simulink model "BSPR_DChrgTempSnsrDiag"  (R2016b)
settings: Solver=FixedStepDiscrete  StartTime=0.0  StopTime=10.0  FixedStep=0.02  RelTol=1e-3  EnableMultiTasking=on
undefined symbols (not defined in the file): BCCR_cntDChrgTempDiag_CW, bin2dec, BSPR_tiDChrgTNegElecMax_C, BSPR_tiDChrgTNegElecMin_C, BSPR_tiDChrgTNegJit_C, BSPR_tiDChrgTNegVld_C, BSPR_tiDChrgTPosElecMax_C, BSPR_tiDChrgTPosElecMin_C, BSPR_tiDChrgTPosJit_C, BSPR_tiDChrgTPosVld_C, BSPR_uDChrgTNegElecMax_C, BSPR_uDChrgTNegElecMin_C, BSPR_uDChrgTNegJitDiff_C, BSPR_uDChrgTPosElecMax_C, BSPR_uDChrgTPosElecMin_C, BSPR_uDChrgTPosJitDiff_C
libraries: simulink x48

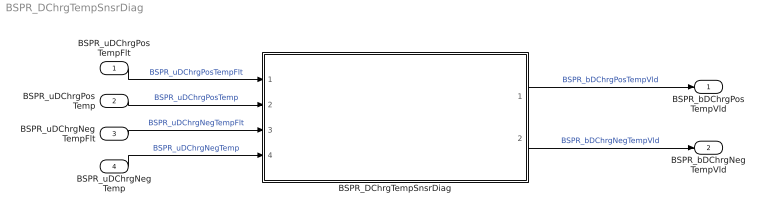
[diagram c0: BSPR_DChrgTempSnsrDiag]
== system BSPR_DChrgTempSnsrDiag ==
  BSPR_uDChrgPosTempFlt : Inport
  BSPR_uDChrgPosTemp : Inport  Port=2
  BSPR_uDChrgNegTempFlt : Inport  Port=3
  BSPR_uDChrgNegTemp : Inport  Port=4
  BSPR_DChrgTempSnsrDiag : Subsystem
  BSPR_bDChrgPosTempVld : Outport
  BSPR_bDChrgNegTempVld : Outport  Port=2
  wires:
  BSPR_uDChrgPosTempFlt/1 -> BSPR_DChrgTempSnsrDiag/1(BSPR_uDChrgPosTempFlt)  "BSPR_uDChrgPosTempFlt"
  BSPR_uDChrgPosTemp/1 -> BSPR_DChrgTempSnsrDiag/2(BSPR_uDChrgPosTemp)  "BSPR_uDChrgPosTemp"
  BSPR_uDChrgNegTempFlt/1 -> BSPR_DChrgTempSnsrDiag/3(BSPR_uDChrgNegTempFlt)  "BSPR_uDChrgNegTempFlt"
  BSPR_uDChrgNegTemp/1 -> BSPR_DChrgTempSnsrDiag/4(BSPR_uDChrgNegTemp)  "BSPR_uDChrgNegTemp"
  BSPR_DChrgTempSnsrDiag/1(BSPR_bDChrgPosTempVld) -> BSPR_bDChrgPosTempVld/1  "BSPR_bDChrgPosTempVld"
  BSPR_DChrgTempSnsrDiag/2(BSPR_bDChrgNegTempVld) -> BSPR_bDChrgNegTempVld/1  "BSPR_bDChrgNegTempVld"

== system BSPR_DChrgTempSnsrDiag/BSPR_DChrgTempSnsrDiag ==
  BSPR_uDChrgPosTempFlt : Inport
  BSPR_uDChrgPosTemp : Inport  Port=2
  BSPR_uDChrgNegTempFlt : Inport  Port=3
  BSPR_uDChrgNegTemp : Inport  Port=4
  DChrgTNegErrChk : Subsystem
  DChrgTPosErrChk : Subsystem
  DChrgTempDsmRpt : Subsystem
  BSPR_bDChrgPosTempVld : Outport
  BSPR_bDChrgNegTempVld : Outport  Port=2
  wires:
  BSPR_uDChrgPosTempFlt/1 -> DChrgTPosErrChk/1(BSPR_uDChrgPosTempFlt)
  BSPR_uDChrgPosTemp/1 -> DChrgTPosErrChk/2(BSPR_uDChrgPosTemp)
  DChrgTPosErrChk/1(BSPR_bDChrgTPosJitErrStt) -> DChrgTempDsmRpt/1(BSPR_bDChrgTPosJitErrStt)
  DChrgTPosErrChk/2(BSPR_bDChrgTPosMaxErrStt) -> DChrgTempDsmRpt/2(BSPR_bDChrgTPosMaxErrStt)
  DChrgTPosErrChk/3(BSPR_bDChrgTPosMinErrStt) -> DChrgTempDsmRpt/3(BSPR_bDChrgTPosMinErrStt)
  DChrgTPosErrChk/4(BSPR_bDChrgTPosJitErrDet) -> DChrgTempDsmRpt/4(BSPR_bDChrgTPosJitErrDet)
  DChrgTPosErrChk/5(BSPR_bDChrgTPosJitErrHeal) -> DChrgTempDsmRpt/5(BSPR_bDChrgTPosJitErrHeal)
  DChrgTPosErrChk/6(BSPR_bDChrgTPosMaxErrDet) -> DChrgTempDsmRpt/6(BSPR_bDChrgTPosMaxErrDet)
  DChrgTPosErrChk/7(BSPR_bDChrgTPosMaxErrHeal) -> DChrgTempDsmRpt/7(BSPR_bDChrgTPosMaxErrHeal)
  DChrgTPosErrChk/8(BSPR_bDChrgTPosMinErrDet) -> DChrgTempDsmRpt/8(BSPR_bDChrgTPosMinErrDet)
  DChrgTPosErrChk/9(BSPR_bDChrgTPosMinErrHeal) -> DChrgTempDsmRpt/9(BSPR_bDChrgTPosMinErrHeal)
  DChrgTempDsmRpt/1(BSPR_bDChrgPosTempVld) -> BSPR_bDChrgPosTempVld/1
  BSPR_uDChrgNegTempFlt/1 -> DChrgTNegErrChk/1(BSPR_uDChrgNegTempFlt)
  BSPR_uDChrgNegTemp/1 -> DChrgTNegErrChk/2(BSPR_uDChrgNegTemp)
  DChrgTempDsmRpt/2(BSPR_bDChrgNegTempVld) -> BSPR_bDChrgNegTempVld/1
  DChrgTNegErrChk/1(BSPR_bDChrgTNegJitErrStt) -> DChrgTempDsmRpt/10(BSPR_bDChrgTNegJitErrStt)
  DChrgTNegErrChk/2(BSPR_bDChrgTNegMaxErrStt) -> DChrgTempDsmRpt/11(BSPR_bDChrgTNegMaxErrStt)
  DChrgTNegErrChk/3(BSPR_bDChrgTNegMinErrStt) -> DChrgTempDsmRpt/12(BSPR_bDChrgTNegMinErrStt)
  DChrgTNegErrChk/4(BSPR_bDChrgTNegJitErrDet) -> DChrgTempDsmRpt/13(BSPR_bDChrgTNegJitErrDet)
  DChrgTNegErrChk/5(BSPR_bDChrgTNegJitErrHeal) -> DChrgTempDsmRpt/14(BSPR_bDChrgTNegJitErrHeal)
  DChrgTNegErrChk/6(BSPR_bDChrgTNegMaxErrDet) -> DChrgTempDsmRpt/15(BSPR_bDChrgTNegMaxErrDet)
  DChrgTNegErrChk/7(BSPR_bDChrgTNegMaxErrHeal) -> DChrgTempDsmRpt/16(BSPR_bDChrgTNegMaxErrHeal)
  DChrgTNegErrChk/8(BSPR_bDChrgTNegMinErrDet) -> DChrgTempDsmRpt/17(BSPR_bDChrgTNegMinErrDet)
  DChrgTNegErrChk/9(BSPR_bDChrgTNegMinErrHeal) -> DChrgTempDsmRpt/18(BSPR_bDChrgTNegMinErrHeal)

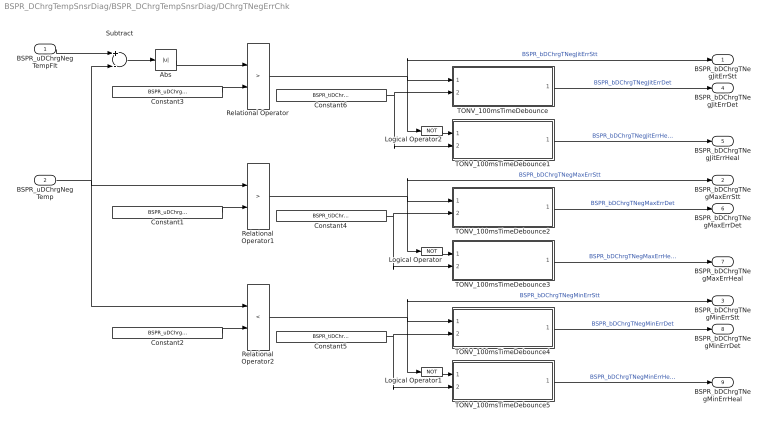
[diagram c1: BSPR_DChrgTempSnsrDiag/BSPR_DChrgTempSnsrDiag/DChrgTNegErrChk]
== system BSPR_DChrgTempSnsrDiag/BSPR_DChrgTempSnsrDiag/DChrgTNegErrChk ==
  BSPR_uDChrgNegTempFlt : Inport
  BSPR_uDChrgNegTemp : Inport  Port=2
  Abs : Abs
  Constant1 : Constant  Value=BSPR_uDChrgTNegElecMax_C  OutDataTypeStr=single
  Constant2 : Constant  Value=BSPR_uDChrgTNegElecMin_C  OutDataTypeStr=single
  Constant3 : Constant  Value=BSPR_uDChrgTNegJitDiff_C  OutDataTypeStr=single
  Constant4 : Constant  Value=BSPR_tiDChrgTNegElecMax_C  OutDataTypeStr=single
  Constant5 : Constant  Value=BSPR_tiDChrgTNegElecMin_C  OutDataTypeStr=single
  Constant6 : Constant  Value=BSPR_tiDChrgTNegJit_C  OutDataTypeStr=single
  Logical Operator : Logic  Operator=NOT  AllPortsSameDT=off  OutDataTypeStr=boolean
  Logical Operator1 : Logic  Operator=NOT  AllPortsSameDT=off  OutDataTypeStr=boolean
  Logical Operator2 : Logic  Operator=NOT  AllPortsSameDT=off  OutDataTypeStr=boolean
  Relational Operator : RelationalOperator  Operator=>  OutDataTypeStr=boolean  RndMeth=Simplest
  Relational Operator1 : RelationalOperator  Operator=>  OutDataTypeStr=boolean  RndMeth=Simplest
  Relational Operator2 : RelationalOperator  Operator=<  OutDataTypeStr=boolean  RndMeth=Simplest
  Subtract : Sum  Inputs=+-
  TONV_100msTimeDebounce : Subsystem  TreatAsAtomicUnit=on  RTWFcnName=TONV_100msTimeDebounce  RTWFileName=SrvLib
  TONV_100msTimeDebounce1 : Subsystem  TreatAsAtomicUnit=on  RTWFcnName=TONV_100msTimeDebounce  RTWFileName=SrvLib
  TONV_100msTimeDebounce2 : Subsystem  TreatAsAtomicUnit=on  RTWFcnName=TONV_100msTimeDebounce  RTWFileName=SrvLib
  TONV_100msTimeDebounce3 : Subsystem  TreatAsAtomicUnit=on  RTWFcnName=TONV_100msTimeDebounce  RTWFileName=SrvLib
  TONV_100msTimeDebounce4 : Subsystem  TreatAsAtomicUnit=on  RTWFcnName=TONV_100msTimeDebounce  RTWFileName=SrvLib
  TONV_100msTimeDebounce5 : Subsystem  TreatAsAtomicUnit=on  RTWFcnName=TONV_100msTimeDebounce  RTWFileName=SrvLib
  BSPR_bDChrgTNegJitErrStt : Outport
  BSPR_bDChrgTNegMaxErrStt : Outport  Port=2
  BSPR_bDChrgTNegMinErrStt : Outport  Port=3
  BSPR_bDChrgTNegJitErrDet : Outport  Port=4
  BSPR_bDChrgTNegJitErrHeal : Outport  Port=5
  BSPR_bDChrgTNegMaxErrDet : Outport  Port=6
  BSPR_bDChrgTNegMaxErrHeal : Outport  Port=7
  BSPR_bDChrgTNegMinErrDet : Outport  Port=8
  BSPR_bDChrgTNegMinErrHeal : Outport  Port=9
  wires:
  TONV_100msTimeDebounce2/1(y) -> BSPR_bDChrgTNegMaxErrDet/1  "BSPR_bDChrgTNegMaxErrDet"
  TONV_100msTimeDebounce1/1(y) -> BSPR_bDChrgTNegJitErrHeal/1  "BSPR_bDChrgTNegJitErrHeal"
  TONV_100msTimeDebounce3/1(y) -> BSPR_bDChrgTNegMaxErrHeal/1  "BSPR_bDChrgTNegMaxErrHeal"
  TONV_100msTimeDebounce4/1(y) -> BSPR_bDChrgTNegMinErrDet/1  "BSPR_bDChrgTNegMinErrDet"
  Logical Operator/1 -> TONV_100msTimeDebounce3/1(u)
  Constant4/1 -> TONV_100msTimeDebounce3/2(T), TONV_100msTimeDebounce2/2(T)
  BSPR_uDChrgNegTemp/1 -> Relational Operator1/1, Relational Operator2/1, Subtract/2
  Relational Operator1/1 -> Logical Operator/1, TONV_100msTimeDebounce2/1(u), BSPR_bDChrgTNegMaxErrStt/1  "BSPR_bDChrgTNegMaxErrStt"
  Constant1/1 -> Relational Operator1/2
  Constant2/1 -> Relational Operator2/2
  Constant6/1 -> TONV_100msTimeDebounce1/2(T), TONV_100msTimeDebounce/2(T)
  Relational Operator/1 -> Logical Operator2/1, TONV_100msTimeDebounce/1(u), BSPR_bDChrgTNegJitErrStt/1  "BSPR_bDChrgTNegJitErrStt"
  BSPR_uDChrgNegTempFlt/1 -> Subtract/1
  Subtract/1 -> Abs/1
  Abs/1 -> Relational Operator/1
  Constant3/1 -> Relational Operator/2
  TONV_100msTimeDebounce/1(y) -> BSPR_bDChrgTNegJitErrDet/1  "BSPR_bDChrgTNegJitErrDet"
  Constant5/1 -> TONV_100msTimeDebounce4/2(T), TONV_100msTimeDebounce5/2(T)
  Relational Operator2/1 -> TONV_100msTimeDebounce4/1(u), Logical Operator1/1, BSPR_bDChrgTNegMinErrStt/1  "BSPR_bDChrgTNegMinErrStt"
  TONV_100msTimeDebounce5/1(y) -> BSPR_bDChrgTNegMinErrHeal/1  "BSPR_bDChrgTNegMinErrHeal"
  Logical Operator1/1 -> TONV_100msTimeDebounce5/1(u)
  Logical Operator2/1 -> TONV_100msTimeDebounce1/1(u)

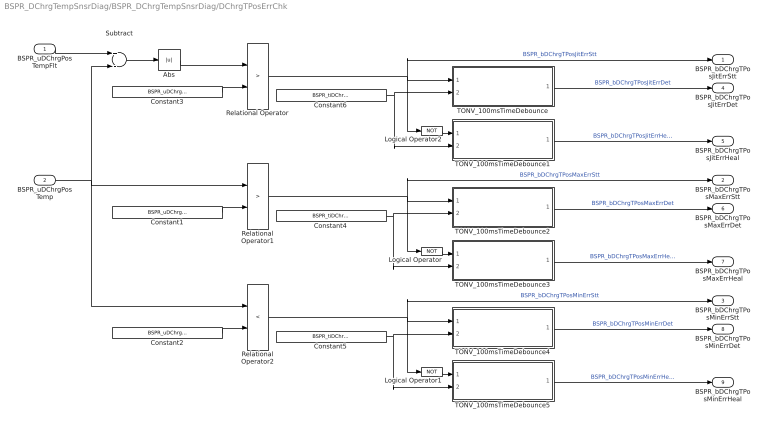
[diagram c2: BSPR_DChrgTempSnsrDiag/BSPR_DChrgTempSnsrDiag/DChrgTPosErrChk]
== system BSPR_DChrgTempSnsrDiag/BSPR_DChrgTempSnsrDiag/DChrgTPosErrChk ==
  BSPR_uDChrgPosTempFlt : Inport
  BSPR_uDChrgPosTemp : Inport  Port=2
  Abs : Abs
  Constant1 : Constant  Value=BSPR_uDChrgTPosElecMax_C  OutDataTypeStr=single
  Constant2 : Constant  Value=BSPR_uDChrgTPosElecMin_C  OutDataTypeStr=single
  Constant3 : Constant  Value=BSPR_uDChrgTPosJitDiff_C  OutDataTypeStr=single
  Constant4 : Constant  Value=BSPR_tiDChrgTPosElecMax_C  OutDataTypeStr=single
  Constant5 : Constant  Value=BSPR_tiDChrgTPosElecMin_C  OutDataTypeStr=single
  Constant6 : Constant  Value=BSPR_tiDChrgTPosJit_C  OutDataTypeStr=single
  Logical Operator : Logic  Operator=NOT  AllPortsSameDT=off  OutDataTypeStr=boolean
  Logical Operator1 : Logic  Operator=NOT  AllPortsSameDT=off  OutDataTypeStr=boolean
  Logical Operator2 : Logic  Operator=NOT  AllPortsSameDT=off  OutDataTypeStr=boolean
  Relational Operator : RelationalOperator  Operator=>  OutDataTypeStr=boolean  RndMeth=Simplest
  Relational Operator1 : RelationalOperator  Operator=>  OutDataTypeStr=boolean  RndMeth=Simplest
  Relational Operator2 : RelationalOperator  Operator=<  OutDataTypeStr=boolean  RndMeth=Simplest
  Subtract : Sum  Inputs=+-
  TONV_100msTimeDebounce : Subsystem  TreatAsAtomicUnit=on  RTWFcnName=TONV_100msTimeDebounce  RTWFileName=SrvLib
  TONV_100msTimeDebounce1 : Subsystem  TreatAsAtomicUnit=on  RTWFcnName=TONV_100msTimeDebounce  RTWFileName=SrvLib
  TONV_100msTimeDebounce2 : Subsystem  TreatAsAtomicUnit=on  RTWFcnName=TONV_100msTimeDebounce  RTWFileName=SrvLib
  TONV_100msTimeDebounce3 : Subsystem  TreatAsAtomicUnit=on  RTWFcnName=TONV_100msTimeDebounce  RTWFileName=SrvLib
  TONV_100msTimeDebounce4 : Subsystem  TreatAsAtomicUnit=on  RTWFcnName=TONV_100msTimeDebounce  RTWFileName=SrvLib
  TONV_100msTimeDebounce5 : Subsystem  TreatAsAtomicUnit=on  RTWFcnName=TONV_100msTimeDebounce  RTWFileName=SrvLib
  BSPR_bDChrgTPosJitErrStt : Outport
  BSPR_bDChrgTPosMaxErrStt : Outport  Port=2
  BSPR_bDChrgTPosMinErrStt : Outport  Port=3
  BSPR_bDChrgTPosJitErrDet : Outport  Port=4
  BSPR_bDChrgTPosJitErrHeal : Outport  Port=5
  BSPR_bDChrgTPosMaxErrDet : Outport  Port=6
  BSPR_bDChrgTPosMaxErrHeal : Outport  Port=7
  BSPR_bDChrgTPosMinErrDet : Outport  Port=8
  BSPR_bDChrgTPosMinErrHeal : Outport  Port=9
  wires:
  Logical Operator1/1 -> TONV_100msTimeDebounce5/1(u)
  TONV_100msTimeDebounce5/1(y) -> BSPR_bDChrgTPosMinErrHeal/1  "BSPR_bDChrgTPosMinErrHeal"
  Relational Operator2/1 -> BSPR_bDChrgTPosMinErrStt/1, Logical Operator1/1, TONV_100msTimeDebounce4/1(u)  "BSPR_bDChrgTPosMinErrStt"
  Constant5/1 -> TONV_100msTimeDebounce5/2(T), TONV_100msTimeDebounce4/2(T)
  TONV_100msTimeDebounce/1(y) -> BSPR_bDChrgTPosJitErrDet/1  "BSPR_bDChrgTPosJitErrDet"
  Constant3/1 -> Relational Operator/2
  Abs/1 -> Relational Operator/1
  Subtract/1 -> Abs/1
  BSPR_uDChrgPosTempFlt/1 -> Subtract/1
  Relational Operator/1 -> Logical Operator2/1, BSPR_bDChrgTPosJitErrStt/1, TONV_100msTimeDebounce/1(u)  "BSPR_bDChrgTPosJitErrStt"
  Constant6/1 -> TONV_100msTimeDebounce/2(T), TONV_100msTimeDebounce1/2(T)
  Constant2/1 -> Relational Operator2/2
  Constant1/1 -> Relational Operator1/2
  Relational Operator1/1 -> BSPR_bDChrgTPosMaxErrStt/1, TONV_100msTimeDebounce2/1(u), Logical Operator/1  "BSPR_bDChrgTPosMaxErrStt"
  BSPR_uDChrgPosTemp/1 -> Subtract/2, Relational Operator2/1, Relational Operator1/1
  Constant4/1 -> TONV_100msTimeDebounce2/2(T), TONV_100msTimeDebounce3/2(T)
  Logical Operator/1 -> TONV_100msTimeDebounce3/1(u)
  TONV_100msTimeDebounce4/1(y) -> BSPR_bDChrgTPosMinErrDet/1  "BSPR_bDChrgTPosMinErrDet"
  TONV_100msTimeDebounce3/1(y) -> BSPR_bDChrgTPosMaxErrHeal/1  "BSPR_bDChrgTPosMaxErrHeal"
  TONV_100msTimeDebounce1/1(y) -> BSPR_bDChrgTPosJitErrHeal/1  "BSPR_bDChrgTPosJitErrHeal"
  TONV_100msTimeDebounce2/1(y) -> BSPR_bDChrgTPosMaxErrDet/1  "BSPR_bDChrgTPosMaxErrDet"
  Logical Operator2/1 -> TONV_100msTimeDebounce1/1(u)

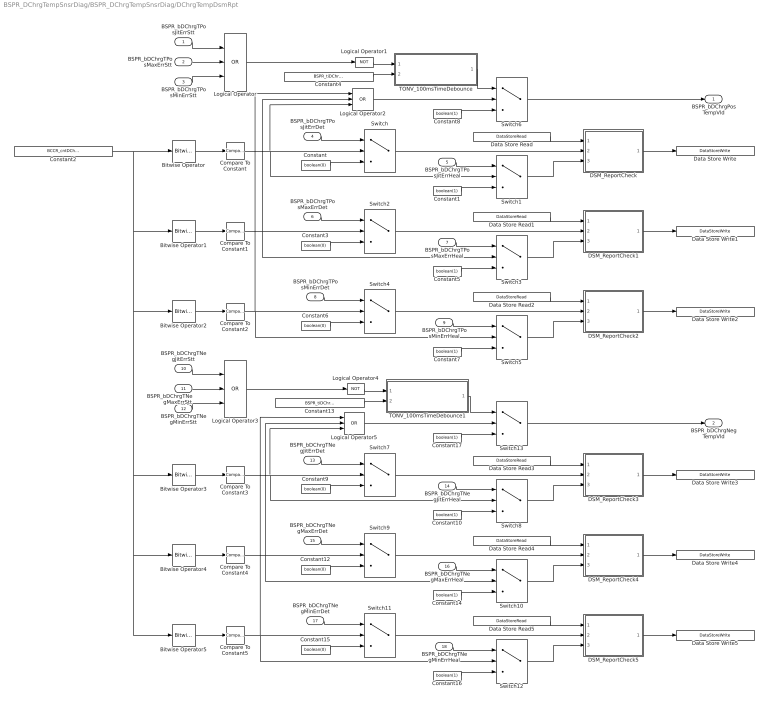
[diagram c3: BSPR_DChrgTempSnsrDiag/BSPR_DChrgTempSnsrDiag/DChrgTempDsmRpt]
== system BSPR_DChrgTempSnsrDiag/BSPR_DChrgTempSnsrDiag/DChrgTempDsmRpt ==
  BSPR_bDChrgTPosJitErrStt : Inport
  BSPR_bDChrgTPosMaxErrStt : Inport  Port=2
  BSPR_bDChrgTPosMinErrStt : Inport  Port=3
  BSPR_bDChrgTPosJitErrDet : Inport  Port=4
  BSPR_bDChrgTPosJitErrHeal : Inport  Port=5
  BSPR_bDChrgTPosMaxErrDet : Inport  Port=6
  BSPR_bDChrgTPosMaxErrHeal : Inport  Port=7
  BSPR_bDChrgTPosMinErrDet : Inport  Port=8
  BSPR_bDChrgTPosMinErrHeal : Inport  Port=9
  BSPR_bDChrgTNegJitErrStt : Inport  Port=10
  BSPR_bDChrgTNegMaxErrStt : Inport  Port=11
  BSPR_bDChrgTNegMinErrStt : Inport  Port=12
  BSPR_bDChrgTNegJitErrDet : Inport  Port=13
  BSPR_bDChrgTNegJitErrHeal : Inport  Port=14
  BSPR_bDChrgTNegMaxErrDet : Inport  Port=15
  BSPR_bDChrgTNegMaxErrHeal : Inport  Port=16
  BSPR_bDChrgTNegMinErrDet : Inport  Port=17
  BSPR_bDChrgTNegMinErrHeal : Inport  Port=18
  Bitwise Operator : simulink/Logic and Bit Operations/Bitwise Operator  logicop=AND  UseBitMask=on  BitMask=bin2dec('00000001')  BitMaskRealWorld=Stored Integer
  Bitwise Operator1 : simulink/Logic and Bit Operations/Bitwise Operator  logicop=AND  UseBitMask=on  BitMask=bin2dec('00000010')  BitMaskRealWorld=Stored Integer
  Bitwise Operator2 : simulink/Logic and Bit Operations/Bitwise Operator  logicop=AND  UseBitMask=on  BitMask=bin2dec('00000100')  BitMaskRealWorld=Stored Integer
  Bitwise Operator3 : simulink/Logic and Bit Operations/Bitwise Operator  logicop=AND  UseBitMask=on  BitMask=bin2dec('00001000')  BitMaskRealWorld=Stored Integer
  Bitwise Operator4 : simulink/Logic and Bit Operations/Bitwise Operator  logicop=AND  UseBitMask=on  BitMask=bin2dec('00010000')  BitMaskRealWorld=Stored Integer
  Bitwise Operator5 : simulink/Logic and Bit Operations/Bitwise Operator  logicop=AND  UseBitMask=on  BitMask=bin2dec('00100000')  BitMaskRealWorld=Stored Integer
  Compare To Constant : simulink/Logic and Bit Operations/Compare To Constant  relop===  const=1  OutDataTypeStr=boolean
  Compare To Constant1 : simulink/Logic and Bit Operations/Compare To Constant  relop===  const=2  OutDataTypeStr=boolean
  Compare To Constant2 : simulink/Logic and Bit Operations/Compare To Constant  relop===  const=4  OutDataTypeStr=boolean
  Compare To Constant3 : simulink/Logic and Bit Operations/Compare To Constant  relop===  const=8  OutDataTypeStr=boolean
  Compare To Constant4 : simulink/Logic and Bit Operations/Compare To Constant  relop===  const=16  OutDataTypeStr=boolean
  Compare To Constant5 : simulink/Logic and Bit Operations/Compare To Constant  relop===  const=32  OutDataTypeStr=boolean
  Constant{,3,6,9,12,15} (6 alike) : Constant  Value=boolean(0)  OutDataTypeStr=boolean
  Constant{1,5,7..8,10,14,16..17} (8 alike) : Constant  Value=boolean(1)  OutDataTypeStr=boolean
  Constant13 : Constant  Value=BSPR_tiDChrgTNegVld_C  OutDataTypeStr=single
  Constant2 : Constant  Value=BCCR_cntDChrgTempDiag_CW
  Constant4 : Constant  Value=BSPR_tiDChrgTPosVld_C  OutDataTypeStr=single
  DSM_ReportCheck : Subsystem  TreatAsAtomicUnit=on  RTWFcnName=DSM_ReportCheck  RTWFileName=SrvLib
  DSM_ReportCheck1 : Subsystem  TreatAsAtomicUnit=on  RTWFcnName=DSM_ReportCheck  RTWFileName=SrvLib
  DSM_ReportCheck2 : Subsystem  TreatAsAtomicUnit=on  RTWFcnName=DSM_ReportCheck  RTWFileName=SrvLib
  DSM_ReportCheck3 : Subsystem  TreatAsAtomicUnit=on  RTWFcnName=DSM_ReportCheck  RTWFileName=SrvLib
  DSM_ReportCheck4 : Subsystem  TreatAsAtomicUnit=on  RTWFcnName=DSM_ReportCheck  RTWFileName=SrvLib
  DSM_ReportCheck5 : Subsystem  TreatAsAtomicUnit=on  RTWFcnName=DSM_ReportCheck  RTWFileName=SrvLib
  Data Store Read : DataStoreRead  DataStoreName=DFC_DChrgTPosElecSig
  Data Store Read1 : DataStoreRead  DataStoreName=DFC_DChrgTPosElecMax
  Data Store Read2 : DataStoreRead  DataStoreName=DFC_DChrgTPosElecMin
  Data Store Read3 : DataStoreRead  DataStoreName=DFC_DChrgTNegElecSig
  Data Store Read4 : DataStoreRead  DataStoreName=DFC_DChrgTNegElecMax
  Data Store Read5 : DataStoreRead  DataStoreName=DFC_DChrgTNegElecMin
  Data Store Write : DataStoreWrite  DataStoreName=DFC_DChrgTPosElecSig
  Data Store Write1 : DataStoreWrite  DataStoreName=DFC_DChrgTPosElecMax
  Data Store Write2 : DataStoreWrite  DataStoreName=DFC_DChrgTPosElecMin
  Data Store Write3 : DataStoreWrite  DataStoreName=DFC_DChrgTNegElecSig
  Data Store Write4 : DataStoreWrite  DataStoreName=DFC_DChrgTNegElecMax
  Data Store Write5 : DataStoreWrite  DataStoreName=DFC_DChrgTNegElecMin
  Logical Operator{,2..3,5} (4 alike) : Logic  Operator=OR  Inputs=3  AllPortsSameDT=off  OutDataTypeStr=boolean
  Logical Operator1 : Logic  Operator=NOT  AllPortsSameDT=off  OutDataTypeStr=boolean
  Logical Operator4 : Logic  Operator=NOT  AllPortsSameDT=off  OutDataTypeStr=boolean
  Switch{,1..13} (14 alike) : Switch  Criteria=u2 > Threshold
  TONV_100msTimeDebounce : Subsystem  TreatAsAtomicUnit=on  RTWFcnName=TONV_100msTimeDebounce  RTWFileName=SrvLib
  TONV_100msTimeDebounce1 : Subsystem  TreatAsAtomicUnit=on  RTWFcnName=TONV_100msTimeDebounce  RTWFileName=SrvLib
  BSPR_bDChrgPosTempVld : Outport
  BSPR_bDChrgNegTempVld : Outport  Port=2
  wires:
  BSPR_bDChrgTPosJitErrStt/1 -> Logical Operator/1
  BSPR_bDChrgTPosMaxErrStt/1 -> Logical Operator/2
  BSPR_bDChrgTPosMinErrStt/1 -> Logical Operator/3
  Logical Operator/1 -> Logical Operator1/1
  Logical Operator1/1 -> TONV_100msTimeDebounce/1(u)
  Switch6/1 -> BSPR_bDChrgPosTempVld/1
  Constant4/1 -> TONV_100msTimeDebounce/2(T)
  Constant/1 -> Switch/3
  BSPR_bDChrgTPosJitErrDet/1 -> Switch/1
  BSPR_bDChrgTPosJitErrHeal/1 -> Switch1/1
  Constant1/1 -> Switch1/3
  Switch1/1 -> DSM_ReportCheck/3(Heal)
  Switch/1 -> DSM_ReportCheck/2(Err)
  Bitwise Operator/1 -> Compare To Constant/1
  Compare To Constant/1 -> Logical Operator2/3, Switch1/2, Switch/2
  Constant3/1 -> Switch2/3
  Constant5/1 -> Switch3/3
  Switch3/1 -> DSM_ReportCheck1/3(Heal)
  Switch2/1 -> DSM_ReportCheck1/2(Err)
  BSPR_bDChrgTPosMaxErrHeal/1 -> Switch3/1
  BSPR_bDChrgTPosMaxErrDet/1 -> Switch2/1
  Bitwise Operator1/1 -> Compare To Constant1/1
  Compare To Constant1/1 -> Switch2/2, Switch3/2, Logical Operator2/2
  Data Store Read1/1 -> DSM_ReportCheck1/1(Dfc_id_nv)
  Data Store Read/1 -> DSM_ReportCheck/1(Dfc_id_nv)
  Constant6/1 -> Switch4/3
  Constant7/1 -> Switch5/3
  Switch5/1 -> DSM_ReportCheck2/3(Heal)
  Switch4/1 -> DSM_ReportCheck2/2(Err)
  BSPR_bDChrgTPosMinErrHeal/1 -> Switch5/1
  BSPR_bDChrgTPosMinErrDet/1 -> Switch4/1
  Bitwise Operator2/1 -> Compare To Constant2/1
  Compare To Constant2/1 -> Switch4/2, Switch5/2, Logical Operator2/1
  Data Store Read2/1 -> DSM_ReportCheck2/1(Dfc_id_nv)
  DSM_ReportCheck/1(Dfc_id) -> Data Store Write/1
  DSM_ReportCheck1/1(Dfc_id) -> Data Store Write1/1
  DSM_ReportCheck2/1(Dfc_id) -> Data Store Write2/1
  TONV_100msTimeDebounce/1(y) -> Switch6/1
  Constant8/1 -> Switch6/3
  Logical Operator2/1 -> Switch6/2
  Constant2/1 -> Bitwise Operator/1, Bitwise Operator1/1, Bitwise Operator2/1, Bitwise Operator3/1, Bitwise Operator4/1, Bitwise Operator5/1
  Logical Operator5/1 -> Switch13/2
  Constant17/1 -> Switch13/3
  TONV_100msTimeDebounce1/1(y) -> Switch13/1
  DSM_ReportCheck5/1(Dfc_id) -> Data Store Write5/1
  DSM_ReportCheck4/1(Dfc_id) -> Data Store Write4/1
  DSM_ReportCheck3/1(Dfc_id) -> Data Store Write3/1
  Data Store Read5/1 -> DSM_ReportCheck5/1(Dfc_id_nv)
  Compare To Constant5/1 -> Switch11/2, Switch12/2, Logical Operator5/1
  Bitwise Operator5/1 -> Compare To Constant5/1
  BSPR_bDChrgTNegMinErrDet/1 -> Switch11/1
  BSPR_bDChrgTNegMinErrHeal/1 -> Switch12/1
  Switch11/1 -> DSM_ReportCheck5/2(Err)
  Switch12/1 -> DSM_ReportCheck5/3(Heal)
  Constant16/1 -> Switch12/3
  Constant15/1 -> Switch11/3
  Data Store Read3/1 -> DSM_ReportCheck3/1(Dfc_id_nv)
  Data Store Read4/1 -> DSM_ReportCheck4/1(Dfc_id_nv)
  Compare To Constant4/1 -> Switch9/2, Switch10/2, Logical Operator5/2
  Bitwise Operator4/1 -> Compare To Constant4/1
  BSPR_bDChrgTNegMaxErrDet/1 -> Switch9/1
  BSPR_bDChrgTNegMaxErrHeal/1 -> Switch10/1
  Switch9/1 -> DSM_ReportCheck4/2(Err)
  Switch10/1 -> DSM_ReportCheck4/3(Heal)
  Constant14/1 -> Switch10/3
  Constant12/1 -> Switch9/3
  Compare To Constant3/1 -> Logical Operator5/3, Switch7/2, Switch8/2
  Bitwise Operator3/1 -> Compare To Constant3/1
  Switch7/1 -> DSM_ReportCheck3/2(Err)
  Switch8/1 -> DSM_ReportCheck3/3(Heal)
  Constant10/1 -> Switch8/3
  BSPR_bDChrgTNegJitErrHeal/1 -> Switch8/1
  BSPR_bDChrgTNegJitErrDet/1 -> Switch7/1
  Constant9/1 -> Switch7/3
  Constant13/1 -> TONV_100msTimeDebounce1/2(T)
  Switch13/1 -> BSPR_bDChrgNegTempVld/1
  Logical Operator4/1 -> TONV_100msTimeDebounce1/1(u)
  Logical Operator3/1 -> Logical Operator4/1
  BSPR_bDChrgTNegMinErrStt/1 -> Logical Operator3/3
  BSPR_bDChrgTNegMaxErrStt/1 -> Logical Operator3/2
  BSPR_bDChrgTNegJitErrStt/1 -> Logical Operator3/1

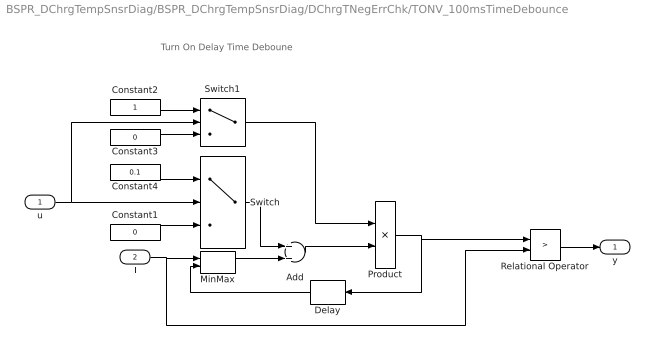
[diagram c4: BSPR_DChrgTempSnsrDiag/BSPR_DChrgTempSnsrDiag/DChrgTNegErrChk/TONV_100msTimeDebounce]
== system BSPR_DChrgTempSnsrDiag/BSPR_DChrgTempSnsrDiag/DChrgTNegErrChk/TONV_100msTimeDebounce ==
  note: Turn On Delay Time Deboune
  u : Inport
  T : Inport  Port=2
  Add : Sum
  Constant1 : Constant  Value=0  OutDataTypeStr=single
  Constant2 : Constant  OutDataTypeStr=uint8
  Constant3 : Constant  Value=0  OutDataTypeStr=uint8
  Constant4 : Constant  Value=0.1  OutDataTypeStr=single
  Delay : Delay  DelayLength=1  InitialCondition=0
  MinMax : MinMax  Inputs=2
  Product : Product  OutMin=[0]  OutMax=[65535]  OutDataTypeStr=single
  Relational Operator : RelationalOperator  Operator=>  OutDataTypeStr=boolean  RndMeth=Simplest
  Switch : Switch  Criteria=u2 ~= 0
  Switch1 : Switch  Criteria=u2 ~= 0
  y : Outport
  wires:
  MinMax/1 -> Add/2
  T/1 -> Relational Operator/2, MinMax/1
  Relational Operator/1 -> y/1
  Delay/1 -> MinMax/2
  Switch/1 -> Add/1
  Product/1 -> Delay/1, Relational Operator/1
  Add/1 -> Product/2
  Constant1/1 -> Switch/3
  Constant4/1 -> Switch/1
  u/1 -> Switch/2, Switch1/2
  Constant2/1 -> Switch1/1
  Constant3/1 -> Switch1/3
  Switch1/1 -> Product/1

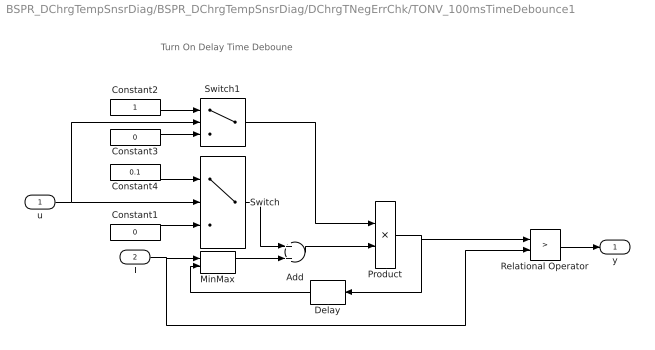
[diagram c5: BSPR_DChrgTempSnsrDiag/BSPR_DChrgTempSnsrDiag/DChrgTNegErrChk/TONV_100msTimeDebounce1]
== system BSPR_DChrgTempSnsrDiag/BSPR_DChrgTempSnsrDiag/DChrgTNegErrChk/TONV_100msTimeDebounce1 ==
  note: Turn On Delay Time Deboune
  u : Inport
  T : Inport  Port=2
  Add : Sum
  Constant1 : Constant  Value=0  OutDataTypeStr=single
  Constant2 : Constant  OutDataTypeStr=uint8
  Constant3 : Constant  Value=0  OutDataTypeStr=uint8
  Constant4 : Constant  Value=0.1  OutDataTypeStr=single
  Delay : Delay  DelayLength=1  InitialCondition=0
  MinMax : MinMax  Inputs=2
  Product : Product  OutMin=[0]  OutMax=[65535]  OutDataTypeStr=single
  Relational Operator : RelationalOperator  Operator=>  OutDataTypeStr=boolean  RndMeth=Simplest
  Switch : Switch  Criteria=u2 ~= 0
  Switch1 : Switch  Criteria=u2 ~= 0
  y : Outport
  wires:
  Switch1/1 -> Product/1
  Constant3/1 -> Switch1/3
  Constant2/1 -> Switch1/1
  u/1 -> Switch1/2, Switch/2
  Constant4/1 -> Switch/1
  Constant1/1 -> Switch/3
  Add/1 -> Product/2
  Product/1 -> Relational Operator/1, Delay/1
  Switch/1 -> Add/1
  Delay/1 -> MinMax/2
  Relational Operator/1 -> y/1
  T/1 -> MinMax/1, Relational Operator/2
  MinMax/1 -> Add/2

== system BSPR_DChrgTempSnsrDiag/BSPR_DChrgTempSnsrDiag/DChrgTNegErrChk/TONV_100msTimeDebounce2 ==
  note: Turn On Delay Time Deboune
  u : Inport
  T : Inport  Port=2
  Add : Sum
  Constant1 : Constant  Value=0  OutDataTypeStr=single
  Constant2 : Constant  OutDataTypeStr=uint8
  Constant3 : Constant  Value=0  OutDataTypeStr=uint8
  Constant4 : Constant  Value=0.1  OutDataTypeStr=single
  Delay : Delay  DelayLength=1  InitialCondition=0
  MinMax : MinMax  Inputs=2
  Product : Product  OutMin=[0]  OutMax=[65535]  OutDataTypeStr=single
  Relational Operator : RelationalOperator  Operator=>  OutDataTypeStr=boolean  RndMeth=Simplest
  Switch : Switch  Criteria=u2 ~= 0
  Switch1 : Switch  Criteria=u2 ~= 0
  y : Outport
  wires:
  Switch1/1 -> Product/1
  Constant3/1 -> Switch1/3
  Constant2/1 -> Switch1/1
  u/1 -> Switch1/2, Switch/2
  Constant4/1 -> Switch/1
  Constant1/1 -> Switch/3
  Add/1 -> Product/2
  Product/1 -> Relational Operator/1, Delay/1
  Switch/1 -> Add/1
  Delay/1 -> MinMax/2
  Relational Operator/1 -> y/1
  T/1 -> MinMax/1, Relational Operator/2
  MinMax/1 -> Add/2

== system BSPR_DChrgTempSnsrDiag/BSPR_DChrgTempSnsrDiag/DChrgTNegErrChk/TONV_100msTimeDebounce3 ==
  note: Turn On Delay Time Deboune
  u : Inport
  T : Inport  Port=2
  Add : Sum
  Constant1 : Constant  Value=0  OutDataTypeStr=single
  Constant2 : Constant  OutDataTypeStr=uint8
  Constant3 : Constant  Value=0  OutDataTypeStr=uint8
  Constant4 : Constant  Value=0.1  OutDataTypeStr=single
  Delay : Delay  DelayLength=1  InitialCondition=0
  MinMax : MinMax  Inputs=2
  Product : Product  OutMin=[0]  OutMax=[65535]  OutDataTypeStr=single
  Relational Operator : RelationalOperator  Operator=>  OutDataTypeStr=boolean  RndMeth=Simplest
  Switch : Switch  Criteria=u2 ~= 0
  Switch1 : Switch  Criteria=u2 ~= 0
  y : Outport
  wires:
  MinMax/1 -> Add/2
  T/1 -> Relational Operator/2, MinMax/1
  Relational Operator/1 -> y/1
  Delay/1 -> MinMax/2
  Switch/1 -> Add/1
  Product/1 -> Delay/1, Relational Operator/1
  Add/1 -> Product/2
  Constant1/1 -> Switch/3
  Constant4/1 -> Switch/1
  u/1 -> Switch/2, Switch1/2
  Constant2/1 -> Switch1/1
  Constant3/1 -> Switch1/3
  Switch1/1 -> Product/1

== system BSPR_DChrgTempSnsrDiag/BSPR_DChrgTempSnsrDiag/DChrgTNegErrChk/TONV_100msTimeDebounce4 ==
  note: Turn On Delay Time Deboune
  u : Inport
  T : Inport  Port=2
  Add : Sum
  Constant1 : Constant  Value=0  OutDataTypeStr=single
  Constant2 : Constant  OutDataTypeStr=uint8
  Constant3 : Constant  Value=0  OutDataTypeStr=uint8
  Constant4 : Constant  Value=0.1  OutDataTypeStr=single
  Delay : Delay  DelayLength=1  InitialCondition=0
  MinMax : MinMax  Inputs=2
  Product : Product  OutMin=[0]  OutMax=[65535]  OutDataTypeStr=single
  Relational Operator : RelationalOperator  Operator=>  OutDataTypeStr=boolean  RndMeth=Simplest
  Switch : Switch  Criteria=u2 ~= 0
  Switch1 : Switch  Criteria=u2 ~= 0
  y : Outport
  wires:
  MinMax/1 -> Add/2
  T/1 -> Relational Operator/2, MinMax/1
  Relational Operator/1 -> y/1
  Delay/1 -> MinMax/2
  Switch/1 -> Add/1
  Product/1 -> Delay/1, Relational Operator/1
  Add/1 -> Product/2
  Constant1/1 -> Switch/3
  Constant4/1 -> Switch/1
  u/1 -> Switch/2, Switch1/2
  Constant2/1 -> Switch1/1
  Constant3/1 -> Switch1/3
  Switch1/1 -> Product/1

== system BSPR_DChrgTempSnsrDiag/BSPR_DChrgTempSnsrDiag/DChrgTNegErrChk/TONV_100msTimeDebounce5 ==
  note: Turn On Delay Time Deboune
  u : Inport
  T : Inport  Port=2
  Add : Sum
  Constant1 : Constant  Value=0  OutDataTypeStr=single
  Constant2 : Constant  OutDataTypeStr=uint8
  Constant3 : Constant  Value=0  OutDataTypeStr=uint8
  Constant4 : Constant  Value=0.1  OutDataTypeStr=single
  Delay : Delay  DelayLength=1  InitialCondition=0
  MinMax : MinMax  Inputs=2
  Product : Product  OutMin=[0]  OutMax=[65535]  OutDataTypeStr=single
  Relational Operator : RelationalOperator  Operator=>  OutDataTypeStr=boolean  RndMeth=Simplest
  Switch : Switch  Criteria=u2 ~= 0
  Switch1 : Switch  Criteria=u2 ~= 0
  y : Outport
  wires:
  Switch1/1 -> Product/1
  Constant3/1 -> Switch1/3
  Constant2/1 -> Switch1/1
  u/1 -> Switch1/2, Switch/2
  Constant4/1 -> Switch/1
  Constant1/1 -> Switch/3
  Add/1 -> Product/2
  Product/1 -> Relational Operator/1, Delay/1
  Switch/1 -> Add/1
  Delay/1 -> MinMax/2
  Relational Operator/1 -> y/1
  T/1 -> MinMax/1, Relational Operator/2
  MinMax/1 -> Add/2

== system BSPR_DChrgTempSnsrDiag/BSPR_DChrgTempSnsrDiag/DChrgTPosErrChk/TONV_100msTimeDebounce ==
  note: Turn On Delay Time Deboune
  u : Inport
  T : Inport  Port=2
  Add : Sum
  Constant1 : Constant  Value=0  OutDataTypeStr=single
  Constant2 : Constant  OutDataTypeStr=uint8
  Constant3 : Constant  Value=0  OutDataTypeStr=uint8
  Constant4 : Constant  Value=0.1  OutDataTypeStr=single
  Delay : Delay  DelayLength=1  InitialCondition=0
  MinMax : MinMax  Inputs=2
  Product : Product  OutMin=[0]  OutMax=[65535]  OutDataTypeStr=single
  Relational Operator : RelationalOperator  Operator=>  OutDataTypeStr=boolean  RndMeth=Simplest
  Switch : Switch  Criteria=u2 ~= 0
  Switch1 : Switch  Criteria=u2 ~= 0
  y : Outport
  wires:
  Switch1/1 -> Product/1
  Constant3/1 -> Switch1/3
  Constant2/1 -> Switch1/1
  u/1 -> Switch1/2, Switch/2
  Constant4/1 -> Switch/1
  Constant1/1 -> Switch/3
  Add/1 -> Product/2
  Product/1 -> Relational Operator/1, Delay/1
  Switch/1 -> Add/1
  Delay/1 -> MinMax/2
  Relational Operator/1 -> y/1
  T/1 -> MinMax/1, Relational Operator/2
  MinMax/1 -> Add/2

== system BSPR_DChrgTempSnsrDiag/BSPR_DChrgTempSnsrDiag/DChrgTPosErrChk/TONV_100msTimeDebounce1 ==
  note: Turn On Delay Time Deboune
  u : Inport
  T : Inport  Port=2
  Add : Sum
  Constant1 : Constant  Value=0  OutDataTypeStr=single
  Constant2 : Constant  OutDataTypeStr=uint8
  Constant3 : Constant  Value=0  OutDataTypeStr=uint8
  Constant4 : Constant  Value=0.1  OutDataTypeStr=single
  Delay : Delay  DelayLength=1  InitialCondition=0
  MinMax : MinMax  Inputs=2
  Product : Product  OutMin=[0]  OutMax=[65535]  OutDataTypeStr=single
  Relational Operator : RelationalOperator  Operator=>  OutDataTypeStr=boolean  RndMeth=Simplest
  Switch : Switch  Criteria=u2 ~= 0
  Switch1 : Switch  Criteria=u2 ~= 0
  y : Outport
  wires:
  MinMax/1 -> Add/2
  T/1 -> Relational Operator/2, MinMax/1
  Relational Operator/1 -> y/1
  Delay/1 -> MinMax/2
  Switch/1 -> Add/1
  Product/1 -> Delay/1, Relational Operator/1
  Add/1 -> Product/2
  Constant1/1 -> Switch/3
  Constant4/1 -> Switch/1
  u/1 -> Switch/2, Switch1/2
  Constant2/1 -> Switch1/1
  Constant3/1 -> Switch1/3
  Switch1/1 -> Product/1

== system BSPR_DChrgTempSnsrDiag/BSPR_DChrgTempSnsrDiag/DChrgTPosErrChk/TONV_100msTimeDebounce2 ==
  note: Turn On Delay Time Deboune
  u : Inport
  T : Inport  Port=2
  Add : Sum
  Constant1 : Constant  Value=0  OutDataTypeStr=single
  Constant2 : Constant  OutDataTypeStr=uint8
  Constant3 : Constant  Value=0  OutDataTypeStr=uint8
  Constant4 : Constant  Value=0.1  OutDataTypeStr=single
  Delay : Delay  DelayLength=1  InitialCondition=0
  MinMax : MinMax  Inputs=2
  Product : Product  OutMin=[0]  OutMax=[65535]  OutDataTypeStr=single
  Relational Operator : RelationalOperator  Operator=>  OutDataTypeStr=boolean  RndMeth=Simplest
  Switch : Switch  Criteria=u2 ~= 0
  Switch1 : Switch  Criteria=u2 ~= 0
  y : Outport
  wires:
  MinMax/1 -> Add/2
  T/1 -> Relational Operator/2, MinMax/1
  Relational Operator/1 -> y/1
  Delay/1 -> MinMax/2
  Switch/1 -> Add/1
  Product/1 -> Delay/1, Relational Operator/1
  Add/1 -> Product/2
  Constant1/1 -> Switch/3
  Constant4/1 -> Switch/1
  u/1 -> Switch/2, Switch1/2
  Constant2/1 -> Switch1/1
  Constant3/1 -> Switch1/3
  Switch1/1 -> Product/1

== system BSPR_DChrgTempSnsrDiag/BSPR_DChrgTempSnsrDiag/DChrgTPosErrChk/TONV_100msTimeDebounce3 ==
  note: Turn On Delay Time Deboune
  u : Inport
  T : Inport  Port=2
  Add : Sum
  Constant1 : Constant  Value=0  OutDataTypeStr=single
  Constant2 : Constant  OutDataTypeStr=uint8
  Constant3 : Constant  Value=0  OutDataTypeStr=uint8
  Constant4 : Constant  Value=0.1  OutDataTypeStr=single
  Delay : Delay  DelayLength=1  InitialCondition=0
  MinMax : MinMax  Inputs=2
  Product : Product  OutMin=[0]  OutMax=[65535]  OutDataTypeStr=single
  Relational Operator : RelationalOperator  Operator=>  OutDataTypeStr=boolean  RndMeth=Simplest
  Switch : Switch  Criteria=u2 ~= 0
  Switch1 : Switch  Criteria=u2 ~= 0
  y : Outport
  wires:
  Switch1/1 -> Product/1
  Constant3/1 -> Switch1/3
  Constant2/1 -> Switch1/1
  u/1 -> Switch1/2, Switch/2
  Constant4/1 -> Switch/1
  Constant1/1 -> Switch/3
  Add/1 -> Product/2
  Product/1 -> Relational Operator/1, Delay/1
  Switch/1 -> Add/1
  Delay/1 -> MinMax/2
  Relational Operator/1 -> y/1
  T/1 -> MinMax/1, Relational Operator/2
  MinMax/1 -> Add/2

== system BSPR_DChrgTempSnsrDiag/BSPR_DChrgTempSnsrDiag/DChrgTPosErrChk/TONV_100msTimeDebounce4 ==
  note: Turn On Delay Time Deboune
  u : Inport
  T : Inport  Port=2
  Add : Sum
  Constant1 : Constant  Value=0  OutDataTypeStr=single
  Constant2 : Constant  OutDataTypeStr=uint8
  Constant3 : Constant  Value=0  OutDataTypeStr=uint8
  Constant4 : Constant  Value=0.1  OutDataTypeStr=single
  Delay : Delay  DelayLength=1  InitialCondition=0
  MinMax : MinMax  Inputs=2
  Product : Product  OutMin=[0]  OutMax=[65535]  OutDataTypeStr=single
  Relational Operator : RelationalOperator  Operator=>  OutDataTypeStr=boolean  RndMeth=Simplest
  Switch : Switch  Criteria=u2 ~= 0
  Switch1 : Switch  Criteria=u2 ~= 0
  y : Outport
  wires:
  Switch1/1 -> Product/1
  Constant3/1 -> Switch1/3
  Constant2/1 -> Switch1/1
  u/1 -> Switch1/2, Switch/2
  Constant4/1 -> Switch/1
  Constant1/1 -> Switch/3
  Add/1 -> Product/2
  Product/1 -> Relational Operator/1, Delay/1
  Switch/1 -> Add/1
  Delay/1 -> MinMax/2
  Relational Operator/1 -> y/1
  T/1 -> MinMax/1, Relational Operator/2
  MinMax/1 -> Add/2

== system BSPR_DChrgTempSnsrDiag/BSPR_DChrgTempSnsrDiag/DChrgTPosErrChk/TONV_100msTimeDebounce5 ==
  note: Turn On Delay Time Deboune
  u : Inport
  T : Inport  Port=2
  Add : Sum
  Constant1 : Constant  Value=0  OutDataTypeStr=single
  Constant2 : Constant  OutDataTypeStr=uint8
  Constant3 : Constant  Value=0  OutDataTypeStr=uint8
  Constant4 : Constant  Value=0.1  OutDataTypeStr=single
  Delay : Delay  DelayLength=1  InitialCondition=0
  MinMax : MinMax  Inputs=2
  Product : Product  OutMin=[0]  OutMax=[65535]  OutDataTypeStr=single
  Relational Operator : RelationalOperator  Operator=>  OutDataTypeStr=boolean  RndMeth=Simplest
  Switch : Switch  Criteria=u2 ~= 0
  Switch1 : Switch  Criteria=u2 ~= 0
  y : Outport
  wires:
  MinMax/1 -> Add/2
  T/1 -> Relational Operator/2, MinMax/1
  Relational Operator/1 -> y/1
  Delay/1 -> MinMax/2
  Switch/1 -> Add/1
  Product/1 -> Delay/1, Relational Operator/1
  Add/1 -> Product/2
  Constant1/1 -> Switch/3
  Constant4/1 -> Switch/1
  u/1 -> Switch/2, Switch1/2
  Constant2/1 -> Switch1/1
  Constant3/1 -> Switch1/3
  Switch1/1 -> Product/1

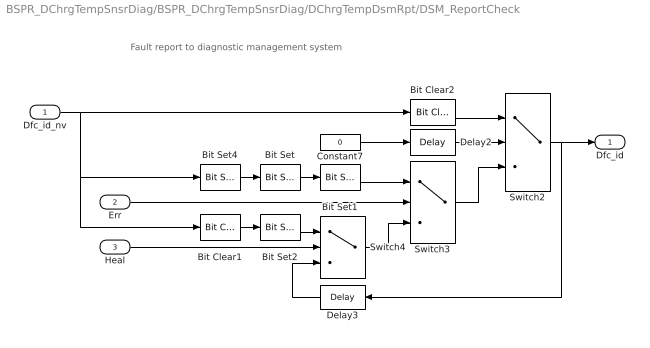
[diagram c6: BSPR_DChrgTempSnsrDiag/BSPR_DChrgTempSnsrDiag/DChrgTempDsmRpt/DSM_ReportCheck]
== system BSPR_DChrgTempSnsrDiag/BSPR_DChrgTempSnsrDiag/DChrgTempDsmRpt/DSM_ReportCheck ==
  note: Fault report to diagnostic management system
  Dfc_id_nv : Inport  OutDataTypeStr=uint8
  Err : Inport  Port=2
  Heal : Inport  Port=3
  Bit Clear1 : simulink/Logic and Bit Operations/Bit Clear  iBit=4
  Bit Clear2 : simulink/Logic and Bit Operations/Bit Clear  iBit=3
  Bit Set : simulink/Logic and Bit Operations/Bit Set  iBit=4
  Bit Set1 : simulink/Logic and Bit Operations/Bit Set  iBit=3
  Bit Set2 : simulink/Logic and Bit Operations/Bit Set  iBit=3
  Bit Set4 : simulink/Logic and Bit Operations/Bit Set  iBit=7
  Constant7 : Constant  Value=0  OutDataTypeStr=boolean
  Delay2 : Delay  DelayLength=1  InitialCondition=1
  Delay3 : Delay  DelayLength=1  InitialCondition=0
  Switch2 : Switch  Criteria=u2 ~= 0
  Switch3 : Switch  Criteria=u2 ~= 0
  Switch4 : Switch  Criteria=u2 ~= 0
  Dfc_id : Outport  OutDataTypeStr=uint8
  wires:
  Dfc_id_nv/1 -> Bit Clear2/1, Bit Set4/1, Bit Clear1/1
  Bit Set4/1 -> Bit Set/1
  Constant7/1 -> Delay2/1
  Delay2/1 -> Switch2/2
  Switch3/1 -> Switch2/3
  Bit Clear2/1 -> Switch2/1
  Switch2/1 -> Delay3/1, Dfc_id/1
  Bit Set1/1 -> Switch3/1
  Bit Set/1 -> Bit Set1/1
  Switch4/1 -> Switch3/3
  Err/1 -> Switch3/2
  Bit Set2/1 -> Switch4/1
  Bit Clear1/1 -> Bit Set2/1
  Delay3/1 -> Switch4/3
  Heal/1 -> Switch4/2

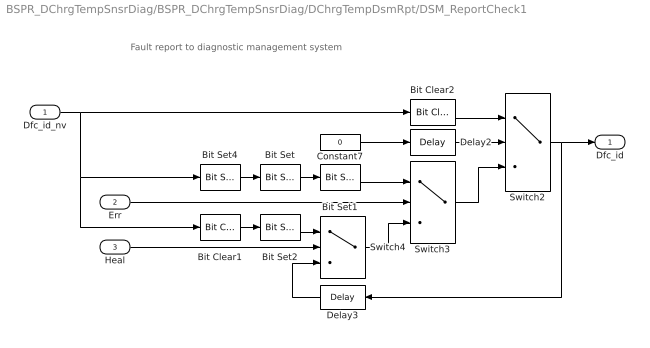
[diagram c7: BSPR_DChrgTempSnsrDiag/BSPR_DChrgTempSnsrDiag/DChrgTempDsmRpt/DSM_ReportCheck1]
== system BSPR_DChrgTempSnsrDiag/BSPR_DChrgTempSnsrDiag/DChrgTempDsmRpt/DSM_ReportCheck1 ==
  note: Fault report to diagnostic management system
  Dfc_id_nv : Inport  OutDataTypeStr=uint8
  Err : Inport  Port=2
  Heal : Inport  Port=3
  Bit Clear1 : simulink/Logic and Bit Operations/Bit Clear  iBit=4
  Bit Clear2 : simulink/Logic and Bit Operations/Bit Clear  iBit=3
  Bit Set : simulink/Logic and Bit Operations/Bit Set  iBit=4
  Bit Set1 : simulink/Logic and Bit Operations/Bit Set  iBit=3
  Bit Set2 : simulink/Logic and Bit Operations/Bit Set  iBit=3
  Bit Set4 : simulink/Logic and Bit Operations/Bit Set  iBit=7
  Constant7 : Constant  Value=0  OutDataTypeStr=boolean
  Delay2 : Delay  DelayLength=1  InitialCondition=1
  Delay3 : Delay  DelayLength=1  InitialCondition=0
  Switch2 : Switch  Criteria=u2 ~= 0
  Switch3 : Switch  Criteria=u2 ~= 0
  Switch4 : Switch  Criteria=u2 ~= 0
  Dfc_id : Outport  OutDataTypeStr=uint8
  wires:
  Heal/1 -> Switch4/2
  Delay3/1 -> Switch4/3
  Bit Clear1/1 -> Bit Set2/1
  Bit Set2/1 -> Switch4/1
  Err/1 -> Switch3/2
  Switch4/1 -> Switch3/3
  Bit Set/1 -> Bit Set1/1
  Bit Set1/1 -> Switch3/1
  Switch2/1 -> Dfc_id/1, Delay3/1
  Bit Clear2/1 -> Switch2/1
  Switch3/1 -> Switch2/3
  Delay2/1 -> Switch2/2
  Constant7/1 -> Delay2/1
  Bit Set4/1 -> Bit Set/1
  Dfc_id_nv/1 -> Bit Clear1/1, Bit Set4/1, Bit Clear2/1

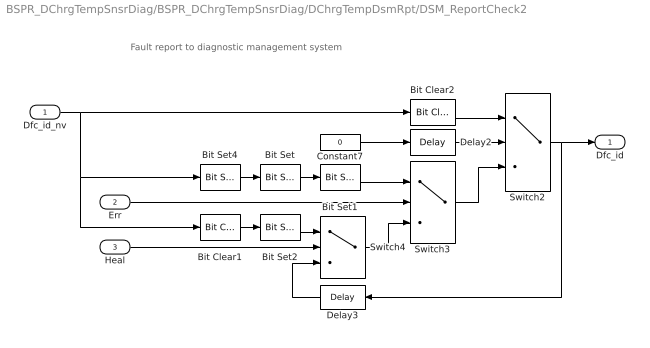
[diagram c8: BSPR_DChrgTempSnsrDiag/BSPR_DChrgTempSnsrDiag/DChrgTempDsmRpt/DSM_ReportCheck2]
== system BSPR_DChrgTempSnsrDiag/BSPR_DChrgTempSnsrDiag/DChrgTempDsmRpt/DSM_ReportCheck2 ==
  note: Fault report to diagnostic management system
  Dfc_id_nv : Inport  OutDataTypeStr=uint8
  Err : Inport  Port=2
  Heal : Inport  Port=3
  Bit Clear1 : simulink/Logic and Bit Operations/Bit Clear  iBit=4
  Bit Clear2 : simulink/Logic and Bit Operations/Bit Clear  iBit=3
  Bit Set : simulink/Logic and Bit Operations/Bit Set  iBit=4
  Bit Set1 : simulink/Logic and Bit Operations/Bit Set  iBit=3
  Bit Set2 : simulink/Logic and Bit Operations/Bit Set  iBit=3
  Bit Set4 : simulink/Logic and Bit Operations/Bit Set  iBit=7
  Constant7 : Constant  Value=0  OutDataTypeStr=boolean
  Delay2 : Delay  DelayLength=1  InitialCondition=1
  Delay3 : Delay  DelayLength=1  InitialCondition=0
  Switch2 : Switch  Criteria=u2 ~= 0
  Switch3 : Switch  Criteria=u2 ~= 0
  Switch4 : Switch  Criteria=u2 ~= 0
  Dfc_id : Outport  OutDataTypeStr=uint8
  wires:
  Dfc_id_nv/1 -> Bit Clear2/1, Bit Set4/1, Bit Clear1/1
  Bit Set4/1 -> Bit Set/1
  Constant7/1 -> Delay2/1
  Delay2/1 -> Switch2/2
  Switch3/1 -> Switch2/3
  Bit Clear2/1 -> Switch2/1
  Switch2/1 -> Delay3/1, Dfc_id/1
  Bit Set1/1 -> Switch3/1
  Bit Set/1 -> Bit Set1/1
  Switch4/1 -> Switch3/3
  Err/1 -> Switch3/2
  Bit Set2/1 -> Switch4/1
  Bit Clear1/1 -> Bit Set2/1
  Delay3/1 -> Switch4/3
  Heal/1 -> Switch4/2

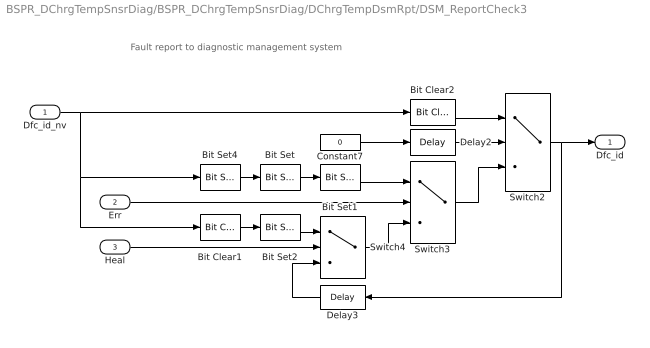
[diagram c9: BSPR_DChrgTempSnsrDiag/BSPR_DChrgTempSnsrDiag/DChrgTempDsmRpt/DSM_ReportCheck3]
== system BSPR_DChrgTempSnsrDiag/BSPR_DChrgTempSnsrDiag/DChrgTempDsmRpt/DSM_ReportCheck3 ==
  note: Fault report to diagnostic management system
  Dfc_id_nv : Inport  OutDataTypeStr=uint8
  Err : Inport  Port=2
  Heal : Inport  Port=3
  Bit Clear1 : simulink/Logic and Bit Operations/Bit Clear  iBit=4
  Bit Clear2 : simulink/Logic and Bit Operations/Bit Clear  iBit=3
  Bit Set : simulink/Logic and Bit Operations/Bit Set  iBit=4
  Bit Set1 : simulink/Logic and Bit Operations/Bit Set  iBit=3
  Bit Set2 : simulink/Logic and Bit Operations/Bit Set  iBit=3
  Bit Set4 : simulink/Logic and Bit Operations/Bit Set  iBit=7
  Constant7 : Constant  Value=0  OutDataTypeStr=boolean
  Delay2 : Delay  DelayLength=1  InitialCondition=1
  Delay3 : Delay  DelayLength=1  InitialCondition=0
  Switch2 : Switch  Criteria=u2 ~= 0
  Switch3 : Switch  Criteria=u2 ~= 0
  Switch4 : Switch  Criteria=u2 ~= 0
  Dfc_id : Outport  OutDataTypeStr=uint8
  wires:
  Heal/1 -> Switch4/2
  Delay3/1 -> Switch4/3
  Bit Clear1/1 -> Bit Set2/1
  Bit Set2/1 -> Switch4/1
  Err/1 -> Switch3/2
  Switch4/1 -> Switch3/3
  Bit Set/1 -> Bit Set1/1
  Bit Set1/1 -> Switch3/1
  Switch2/1 -> Dfc_id/1, Delay3/1
  Bit Clear2/1 -> Switch2/1
  Switch3/1 -> Switch2/3
  Delay2/1 -> Switch2/2
  Constant7/1 -> Delay2/1
  Bit Set4/1 -> Bit Set/1
  Dfc_id_nv/1 -> Bit Clear1/1, Bit Set4/1, Bit Clear2/1

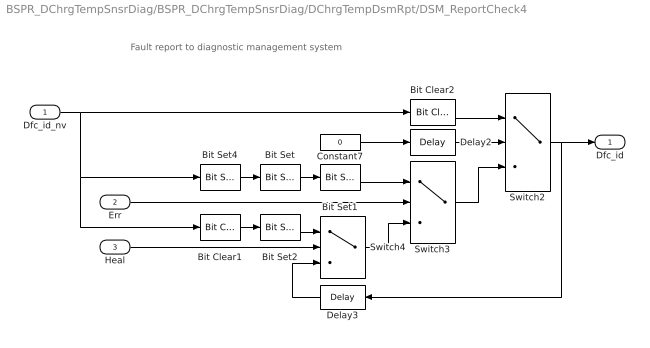
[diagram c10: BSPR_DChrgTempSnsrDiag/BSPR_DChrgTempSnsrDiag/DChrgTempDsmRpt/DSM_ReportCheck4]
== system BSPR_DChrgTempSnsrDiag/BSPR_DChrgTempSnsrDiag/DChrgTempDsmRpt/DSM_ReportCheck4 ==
  note: Fault report to diagnostic management system
  Dfc_id_nv : Inport  OutDataTypeStr=uint8
  Err : Inport  Port=2
  Heal : Inport  Port=3
  Bit Clear1 : simulink/Logic and Bit Operations/Bit Clear  iBit=4
  Bit Clear2 : simulink/Logic and Bit Operations/Bit Clear  iBit=3
  Bit Set : simulink/Logic and Bit Operations/Bit Set  iBit=4
  Bit Set1 : simulink/Logic and Bit Operations/Bit Set  iBit=3
  Bit Set2 : simulink/Logic and Bit Operations/Bit Set  iBit=3
  Bit Set4 : simulink/Logic and Bit Operations/Bit Set  iBit=7
  Constant7 : Constant  Value=0  OutDataTypeStr=boolean
  Delay2 : Delay  DelayLength=1  InitialCondition=1
  Delay3 : Delay  DelayLength=1  InitialCondition=0
  Switch2 : Switch  Criteria=u2 ~= 0
  Switch3 : Switch  Criteria=u2 ~= 0
  Switch4 : Switch  Criteria=u2 ~= 0
  Dfc_id : Outport  OutDataTypeStr=uint8
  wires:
  Dfc_id_nv/1 -> Bit Clear2/1, Bit Set4/1, Bit Clear1/1
  Bit Set4/1 -> Bit Set/1
  Constant7/1 -> Delay2/1
  Delay2/1 -> Switch2/2
  Switch3/1 -> Switch2/3
  Bit Clear2/1 -> Switch2/1
  Switch2/1 -> Delay3/1, Dfc_id/1
  Bit Set1/1 -> Switch3/1
  Bit Set/1 -> Bit Set1/1
  Switch4/1 -> Switch3/3
  Err/1 -> Switch3/2
  Bit Set2/1 -> Switch4/1
  Bit Clear1/1 -> Bit Set2/1
  Delay3/1 -> Switch4/3
  Heal/1 -> Switch4/2

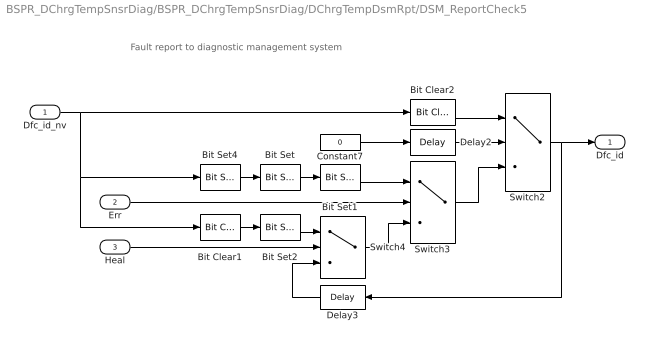
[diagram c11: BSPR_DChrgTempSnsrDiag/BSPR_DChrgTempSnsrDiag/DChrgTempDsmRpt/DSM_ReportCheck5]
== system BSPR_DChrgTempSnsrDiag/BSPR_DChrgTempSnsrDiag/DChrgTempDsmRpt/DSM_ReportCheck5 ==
  note: Fault report to diagnostic management system
  Dfc_id_nv : Inport  OutDataTypeStr=uint8
  Err : Inport  Port=2
  Heal : Inport  Port=3
  Bit Clear1 : simulink/Logic and Bit Operations/Bit Clear  iBit=4
  Bit Clear2 : simulink/Logic and Bit Operations/Bit Clear  iBit=3
  Bit Set : simulink/Logic and Bit Operations/Bit Set  iBit=4
  Bit Set1 : simulink/Logic and Bit Operations/Bit Set  iBit=3
  Bit Set2 : simulink/Logic and Bit Operations/Bit Set  iBit=3
  Bit Set4 : simulink/Logic and Bit Operations/Bit Set  iBit=7
  Constant7 : Constant  Value=0  OutDataTypeStr=boolean
  Delay2 : Delay  DelayLength=1  InitialCondition=1
  Delay3 : Delay  DelayLength=1  InitialCondition=0
  Switch2 : Switch  Criteria=u2 ~= 0
  Switch3 : Switch  Criteria=u2 ~= 0
  Switch4 : Switch  Criteria=u2 ~= 0
  Dfc_id : Outport  OutDataTypeStr=uint8
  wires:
  Heal/1 -> Switch4/2
  Delay3/1 -> Switch4/3
  Bit Clear1/1 -> Bit Set2/1
  Bit Set2/1 -> Switch4/1
  Err/1 -> Switch3/2
  Switch4/1 -> Switch3/3
  Bit Set/1 -> Bit Set1/1
  Bit Set1/1 -> Switch3/1
  Switch2/1 -> Dfc_id/1, Delay3/1
  Bit Clear2/1 -> Switch2/1
  Switch3/1 -> Switch2/3
  Delay2/1 -> Switch2/2
  Constant7/1 -> Delay2/1
  Bit Set4/1 -> Bit Set/1
  Dfc_id_nv/1 -> Bit Clear1/1, Bit Set4/1, Bit Clear2/1

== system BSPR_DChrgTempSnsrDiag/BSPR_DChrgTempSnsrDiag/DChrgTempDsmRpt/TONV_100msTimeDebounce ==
  note: Turn On Delay Time Deboune
  u : Inport
  T : Inport  Port=2
  Add : Sum
  Constant1 : Constant  Value=0  OutDataTypeStr=single
  Constant2 : Constant  OutDataTypeStr=uint8
  Constant3 : Constant  Value=0  OutDataTypeStr=uint8
  Constant4 : Constant  Value=0.1  OutDataTypeStr=single
  Delay : Delay  DelayLength=1  InitialCondition=0
  MinMax : MinMax  Inputs=2
  Product : Product  OutMin=[0]  OutMax=[65535]  OutDataTypeStr=single
  Relational Operator : RelationalOperator  Operator=>  OutDataTypeStr=boolean  RndMeth=Simplest
  Switch : Switch  Criteria=u2 ~= 0
  Switch1 : Switch  Criteria=u2 ~= 0
  y : Outport
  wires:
  Switch1/1 -> Product/1
  Constant3/1 -> Switch1/3
  Constant2/1 -> Switch1/1
  u/1 -> Switch1/2, Switch/2
  Constant4/1 -> Switch/1
  Constant1/1 -> Switch/3
  Add/1 -> Product/2
  Product/1 -> Relational Operator/1, Delay/1
  Switch/1 -> Add/1
  Delay/1 -> MinMax/2
  Relational Operator/1 -> y/1
  T/1 -> MinMax/1, Relational Operator/2
  MinMax/1 -> Add/2

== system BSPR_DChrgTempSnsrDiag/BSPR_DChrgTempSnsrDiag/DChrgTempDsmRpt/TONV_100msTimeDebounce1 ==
  note: Turn On Delay Time Deboune
  u : Inport
  T : Inport  Port=2
  Add : Sum
  Constant1 : Constant  Value=0  OutDataTypeStr=single
  Constant2 : Constant  OutDataTypeStr=uint8
  Constant3 : Constant  Value=0  OutDataTypeStr=uint8
  Constant4 : Constant  Value=0.1  OutDataTypeStr=single
  Delay : Delay  DelayLength=1  InitialCondition=0
  MinMax : MinMax  Inputs=2
  Product : Product  OutMin=[0]  OutMax=[65535]  OutDataTypeStr=single
  Relational Operator : RelationalOperator  Operator=>  OutDataTypeStr=boolean  RndMeth=Simplest
  Switch : Switch  Criteria=u2 ~= 0
  Switch1 : Switch  Criteria=u2 ~= 0
  y : Outport
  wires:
  MinMax/1 -> Add/2
  T/1 -> Relational Operator/2, MinMax/1
  Relational Operator/1 -> y/1
  Delay/1 -> MinMax/2
  Switch/1 -> Add/1
  Product/1 -> Delay/1, Relational Operator/1
  Add/1 -> Product/2
  Constant1/1 -> Switch/3
  Constant4/1 -> Switch/1
  u/1 -> Switch/2, Switch1/2
  Constant2/1 -> Switch1/1
  Constant3/1 -> Switch1/3
  Switch1/1 -> Product/1
